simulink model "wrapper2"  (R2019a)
settings: Solver=VariableStepAuto  StartTime=0.0  StopTime=10.0  RelTol=1e-3
undefined symbols (not defined in the file or in its folder): signal1, signal2, signal3, signal4

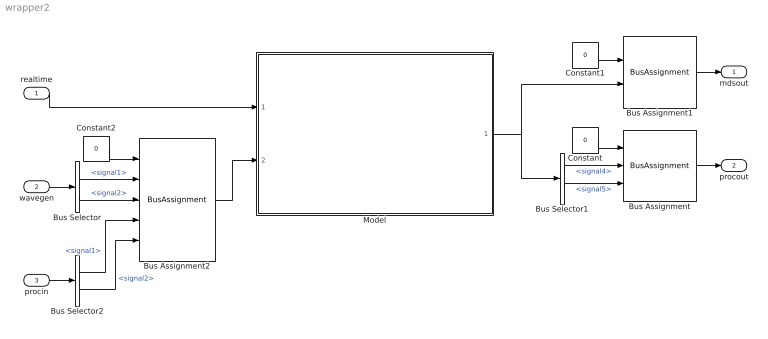
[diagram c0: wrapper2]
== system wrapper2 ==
  realtime : Inport
  wavegen : Inport  Port=2  OutDataTypeStr=Bus: WG0602bus
  procin : Inport  Port=3  OutDataTypeStr=Bus: procin
  Bus Assignment : BusAssignment  AssignedSignals=signal1,signal2
  Bus Assignment1 : BusAssignment  AssignedSignals=cfs2
  Bus Assignment2 : BusAssignment  AssignedSignals=signal1,signal2,signal3,signal4
  Bus Selector : BusSelector  OutputSignals=signal1,signal2
  Bus Selector1 : BusSelector  OutputSignals=signal4,signal5
  Bus Selector2 : BusSelector  OutputSignals=proc01.signal1,proc01.signal2
  Constant : Constant  Value=0  OutDataTypeStr=Bus: procout02
  Constant1 : Constant  Value=0  OutDataTypeStr=Bus: mdsout02
  Constant2 : Constant  Value=0  OutDataTypeStr=Bus: algo_cfs2_inBus
  Model : ModelReference  ModelNameDialog=algo_cfs2.slx  SimulationMode=Normal  ModelReferenceVersion=1.796  SimulationMode=Normal
  mdsout : Outport  OutDataTypeStr=Bus: mdsout02
  procout : Outport  Port=2  OutDataTypeStr=Bus: procout02
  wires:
  realtime/1 -> Model/1
  Constant/1 -> Bus Assignment/1
  Bus Selector1/1 -> Bus Assignment/2  "<signal4>"
  Bus Selector1/2 -> Bus Assignment/3  "<signal5>"
  Bus Assignment1/1 -> mdsout/1
  Model/1 -> Bus Assignment1/2, Bus Selector1/1
  Bus Assignment/1 -> procout/1
  Constant1/1 -> Bus Assignment1/1
  Bus Selector/1 -> Bus Assignment2/2  "<signal1>"
  Bus Selector/2 -> Bus Assignment2/3  "<signal2>"
  wavegen/1 -> Bus Selector/1
  Bus Assignment2/1 -> Model/2
  Constant2/1 -> Bus Assignment2/1
  procin/1 -> Bus Selector2/1
  Bus Selector2/1 -> Bus Assignment2/4  "<signal1>"
  Bus Selector2/2 -> Bus Assignment2/5  "<signal2>"
